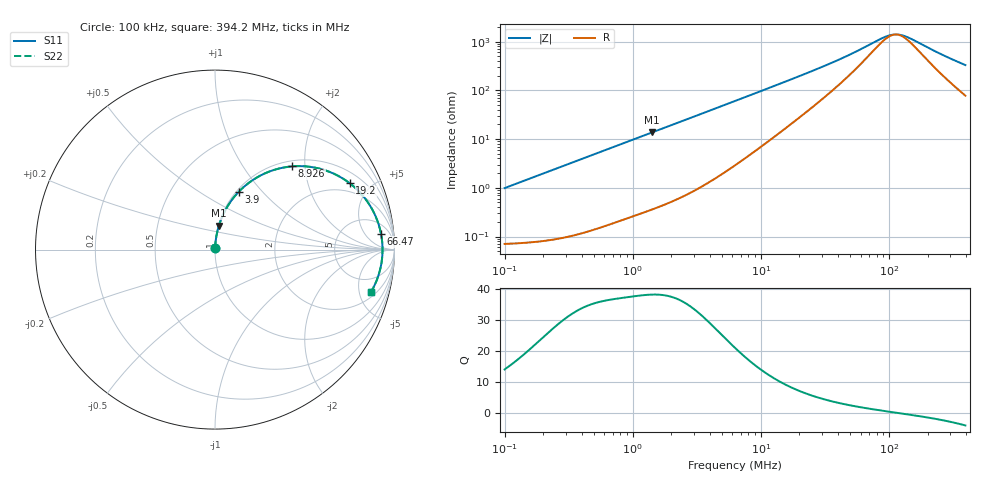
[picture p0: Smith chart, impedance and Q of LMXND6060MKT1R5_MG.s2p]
! LMXND6060MKT1R5_MG  S-PARAMETER MODEL  ( General Type )
! Model Generated by TAIYO YUDEN Corporation (http://www.ty-top.com)
! Version 1.0
! TAIYO YUDEN Control No. 191025NI43SB-FBB
! Copyright(c) 2019 TAIYO YUDEN CO.,LTD. All Rights Reserved.
! Product Description (link to TY-COMPAS)
! https://ds.yuden.co.jp/TYCOMPAS/or/detail?pn=LMXND6060MKT1R5NMG&u=M
! Products Name : Inductors
! Characteristics :
!  Inductance : 1.5 uH , SRF(min) : 69 MHz , DC Resistance(max) : 0.0804 Ohm
!  Rated Current : Saturation :2600 mA , Temp Rise : 2100 mA
!  Case Size : 6.0 x 6.0 / 0.236 x 0.236 [mm/inch] , Thickness : 1.2 / 0.047 [mm/inch]
!  (Conditions: Temperature = 25 degC , DC Bias Current/Voltage = 0A / 0V)
! External Node Assignments :
!  1  o---GGG---o  2
! GND o---------o GND
! Frequency Range : 0.1MHz  -  394.189695MHz  [ 402 STEP ]
# MHz S RI R 50
! Freq[MHz].  S11 Real  S11 Imag  S21 Real  S21 Imag  S12 Real  S12 Imag  S22 Real  S22 Imag
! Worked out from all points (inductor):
!   401 points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, 100 kHz to 394.2 MHz, reference 50 ohm
!   read as one part in series: L = 1.57 uH near 104.2 kHz
!   highest Q = 38.1 at 1.415 MHz (marker M1), where L = 1.54 uH
!   self-resonance near 113.1 MHz
!   S11 on the Smith chart (normalised r, x): 100 kHz: 1.00, +0.02; 3.9 MHz: 1.03, +0.75; 8.926 MHz: 1.11, +1.72; 19.2 MHz: 1.51, +3.73; 66.47 MHz: 10, +13; 394.2 MHz: 2.55, -6.41
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0.1  0.000802 0.00984  0.9992 -0.00984  0.9992 -0.00984  0.000802 0.00984
0.400203  0.0027 0.0391  0.9973 -0.0391  0.9973 -0.0391  0.0027 0.0391
0.792367  0.00797 0.0764  0.992 -0.0764  0.992 -0.0764  0.00797 0.0764
1.414574  0.0217 0.1333  0.9783 -0.1333  0.9783 -0.1333  0.0217 0.1333
1.601627  0.0271 0.1499  0.9729 -0.1499  0.9729 -0.1499  0.0271 0.1499
2.632107  0.0663 0.2349  0.9337 -0.2349  0.9337 -0.2349  0.0663 0.2349
3.900314  0.1317 0.3215  0.8683 -0.3215  0.8683 -0.3215  0.1317 0.3215
5.000008  0.1974 0.3785  0.8026 -0.3785  0.8026 -0.3785  0.1974 0.3785
6.278453  0.277 0.4243  0.723 -0.4243  0.723 -0.4243  0.277 0.4243
8.926272  0.4302 0.4637  0.5698 -0.4637  0.5698 -0.4637  0.4302 0.4637
12.69076  0.5936 0.4481  0.4064 -0.4481  0.4064 -0.4481  0.5936 0.4481
19.19874  0.7514 0.3691  0.2486 -0.3691  0.2486 -0.3691  0.7514 0.3691
25.12657  0.822 0.3021  0.178 -0.3021  0.178 -0.3021  0.822 0.3021
32.21102  0.8666 0.2402  0.1334 -0.2402  0.1334 -0.2402  0.8666 0.2402
42.15653  0.8979 0.1782  0.1021 -0.1782  0.1021 -0.1782  0.8979 0.1782
66.47045  0.9249 0.0885  0.0751 -0.0885  0.0751 -0.0885  0.9249 0.0885
86.99395  0.9315 0.0425  0.0685 -0.0425  0.0685 -0.0425  0.9315 0.0425
100.5574  0.933 0.0189  0.067 -0.0189  0.067 -0.0189  0.933 0.0189
116.2355  0.9334 -0.00439  0.0666 0.00439  0.0666 0.00439  0.9334 -0.00439
134.358  0.9326 -0.0278  0.0674 0.0278  0.0674 0.0278  0.9326 -0.0278
260.5674  0.9099 -0.1462  0.0901 0.1462  0.0901 0.1462  0.9099 -0.1462
394.1897  0.8678 -0.2386  0.1322 0.2386  0.1322 0.2386  0.8678 -0.2386
